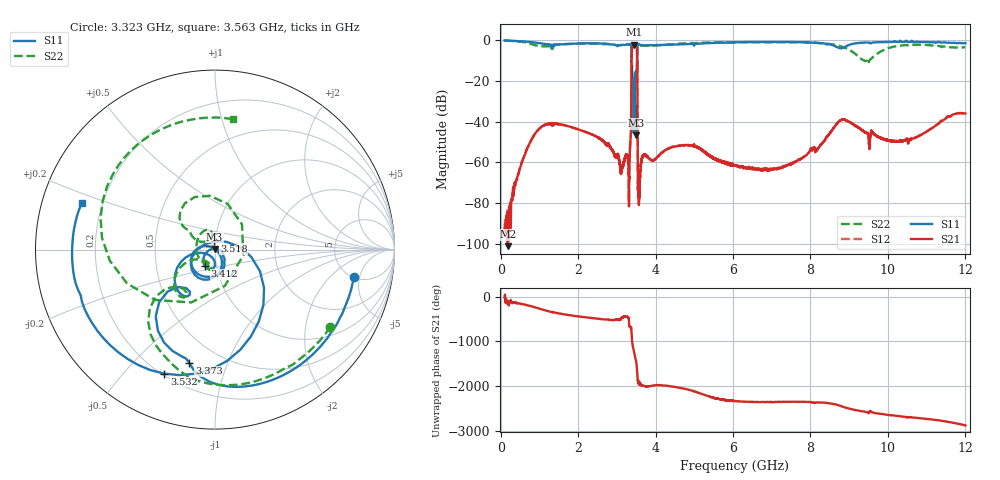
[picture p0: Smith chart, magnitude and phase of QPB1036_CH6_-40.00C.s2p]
! TDS: K:\Engsetup\Winsaw\QPB1036_ALL
! Channel 1
! Ports=1 2
! seg 1=100.000000 1100.000000 101
! seg 2=1101.000000 1501.000000 401
! seg 3=1502.000000 2502.000000 101
! seg 4=2503.000000 3803.000000 1301
! seg 5=3804.000000 5004.000000 121
! seg 6=5005.000000 6005.000000 1001
! seg 7=6006.000000 8406.000000 241
! seg 8=8407.000000 10607.000000 2201
! seg 9=10608.000000 12008.000000 141
! Points=5609
! FailCode=0
! Topology=ALL_SE(12)
!VNA Cal loaded =QPB1036_ALL_-40C
!PS1(V)= 5.000
!PS(mA)= 0.800
!PS2(V)= 1.170
!PS(mA)= -0.100
!PS3(V)= 1.170
!PS(mA)= 0.100
!PS4(V)= 0.630
!PS(mA)= -0.100
!Temp (C)= -40.00
# MHz S DB R 50
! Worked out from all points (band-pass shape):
!   5609 points, 100 MHz to 12.01 GHz, reference 50 ohm
!   highest |S21| = -2.34 dB at 3.444 GHz (marker M1); lowest = -101.0 dB at 180 MHz (marker M2)
!   |S21| within 3 dB of the highest: 3.389 GHz to 3.521 GHz (131.6 MHz wide, 3.81 % of centre)
!   lowest |S11| = -46.6 dB at 3.499 GHz (marker M3), VSWR 1.01, Z = 49.8 + j0.416 ohm
!   |S11| at or under -10 dB: 3.382 GHz to 3.523 GHz (141 MHz wide, 4.08 % of centre)
!   |S22| runs from -24.0 to -0.3 dB; largest |S21 - S12| = 0.008
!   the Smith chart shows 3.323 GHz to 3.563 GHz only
!   S11 on the Smith chart (normalised r, x): 3.323 GHz: 5.08, -4.08; 3.373 GHz: 0.34, -0.74; 3.412 GHz: 0.88, -0.16; 3.518 GHz: 0.99, +0.09; 3.532 GHz: 0.21, -0.65; 3.563 GHz: 0.12, +0.17
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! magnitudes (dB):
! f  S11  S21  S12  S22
! 100 MHz  -0.2  -93.5  -95.7  -0.3
! 180 MHz  -0.3  -101.0  -83.7  -0.3
! 1.124 GHz  -1.9  -41.7  -41.7  -3.1
! 2.092 GHz  -1.7  -44.4  -44.3  -1.8
! 3.323 GHz  -2.1  -63.4  -63.1  -2.2
! 3.342 GHz  -2.0  -52.0  -52.3  -2.2
! 3.373 GHz  -3.8  -26.2  -26.3  -3.3
! 3.412 GHz  -19.3  -2.8  -2.8  -18.8
! 3.444 GHz  -24.9  -2.3  -2.3  -20.2
! 3.499 GHz  -46.6  -2.9  -2.9  -23.9
! 3.518 GHz  -26.7  -4.5  -4.5  -13.1
! 3.532 GHz  -2.5  -25.7  -25.6  -4.6
! 3.563 GHz  -2.1  -71.4  -72.6  -2.7
! 3.678 GHz  -2.6  -56.5  -56.7  -2.8
! 4.074 GHz  -2.5  -57.0  -56.8  -2.7
! 5.004 GHz  -2.1  -52.3  -52.3  -1.6
! 6.056 GHz  -1.1  -61.4  -61.5  -1.2
! 8.046 GHz  -1.3  -54.3  -54.3  -1.3
! 8.829 GHz  -3.9  -39.1  -39.1  -3.3
! 9.495 GHz  -1.2  -45.7  -45.7  -10.9
! 10.02 GHz  -0.9  -49.2  -49.3  -4.0
! 12.01 GHz  -1.5  -36.1  -36.1  -3.5
